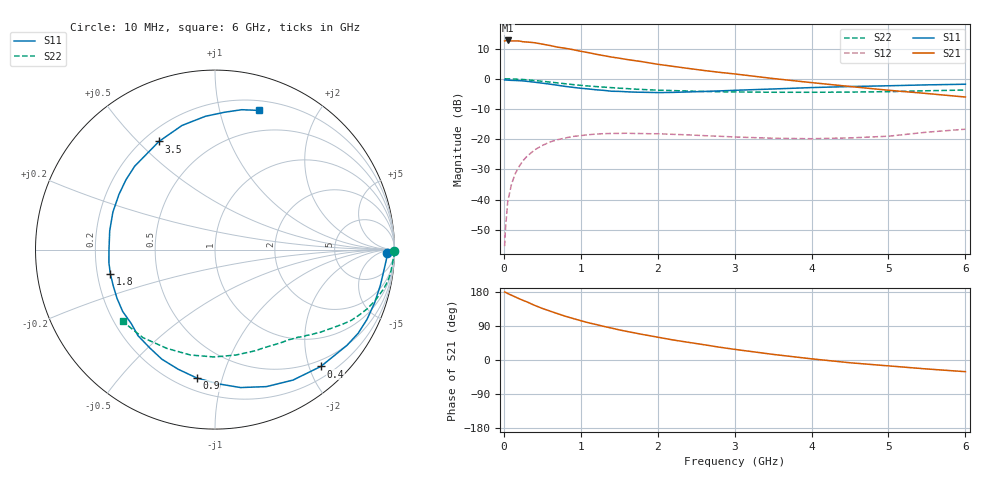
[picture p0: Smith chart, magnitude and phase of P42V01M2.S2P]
! SIEMENS Small Signal Semiconductors
! BFP182
! Si NPN RF Bipolar Junction Transistor in SOT143
! VCE = 2 V  IC = 1.2 mA
! Common Emitter S-Parameters:  March  1996
# GHz  S  MA  R  50
!  f  S11  S21  S12  S22
! GHz  MAG  ANG  MAG  ANG  MAG  ANG  MAG  ANG
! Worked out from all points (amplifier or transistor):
!   36 points, 10 MHz to 6 GHz, reference 50 ohm
!   highest |S21| = 12.7 dB at 50 MHz (marker M1)
!   |S21| within 3 dB of that: start of sweep to 890.3 MHz
!   unconditionally stable (mu >= 1): 2.509 GHz to end of sweep
!   at 250 MHz: K = 0.10, MSG = 19.7 dB, |S12| = -27.1 dB
!   at 1.4 GHz: K = 0.57, MSG = 12.6 dB, |S12| = -18.1 dB
!   at 6 GHz: K = 1.05, MAG = 4.0 dB, |S12| = -16.7 dB
!   S11 on the Smith chart (normalised r, x): 10 MHz: 37, -17; 400 MHz: 0.39, -2.20; 900 MHz: 0.28, -0.83; 1.8 GHz: 0.25, -0.11; 3.5 GHz: 0.26, +0.58; 6 GHz: 0.29, +1.32
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0.01  0.956 -1.2  4.224 179.5  0.0017 84.7  0.999 -0.5
0.02  0.959 -2.4  4.279 178.9  0.0031 89.0  0.9999 -0.9
0.05  0.9494 -6.3  4.31 175.5  0.0092 90.1  0.997 -2.3
0.1  0.9426 -12.2  4.225 170.9  0.0182 81.6  0.9911 -4.7
0.15  0.9374 -18.4  4.232 166.3  0.0272 78.6  0.9876 -7.0
0.2  0.9318 -24.7  4.222 161.6  0.0357 75.0  0.982 -9.3
0.4  0.8785 -47.8  3.953 144.2  0.0666 61.1  0.9369 -17.6
0.5  0.847 -59.1  3.748 136.1  0.0788 54.7  0.9095 -21.3
0.6  0.8155 -69.4  3.554 129.1  0.0901 49.2  0.8823 -24.4
0.8  0.7476 -88.8  3.197 115.5  0.105 39.0  0.8279 -29.9
0.9  0.722 -98.2  3.036 109.5  0.1112 34.8  0.802 -32.2
1.1  0.6786 -115.9  2.709 98.3  0.1188 27.2  0.7601 -36.4
1.3  0.6435 -131.8  2.416 88.7  0.1237 21.1  0.7281 -39.9
1.5  0.6192 -146.2  2.194 79.5  0.1249 16.0  0.6994 -43.1
1.8  0.5985 -167.0  1.917 67.5  0.1242 10.3  0.6657 -47.6
2.2  0.5959 169.9  1.607 52.9  0.1204 4.5  0.6381 -54.0
2.8  0.6304 141.9  1.281 33.9  0.112 0.6  0.6099 -64.4
3.5  0.6785 117.4  1.011 14.8  0.1037 1.1  0.5988 -78.7
4  0.7157 104.9  0.865 3.1  0.102 5.1  0.5982 -90.5
4.5  0.7447 94.1  0.746 -7.3  0.1052 8.9  0.603 -103.1
5.5  0.7935 79.2  0.571 -23.7  0.1309 15.5  0.6339 -129.3
6  0.8131 72.5  0.499 -30.8  0.1465 13.9  0.6516 -142.1
